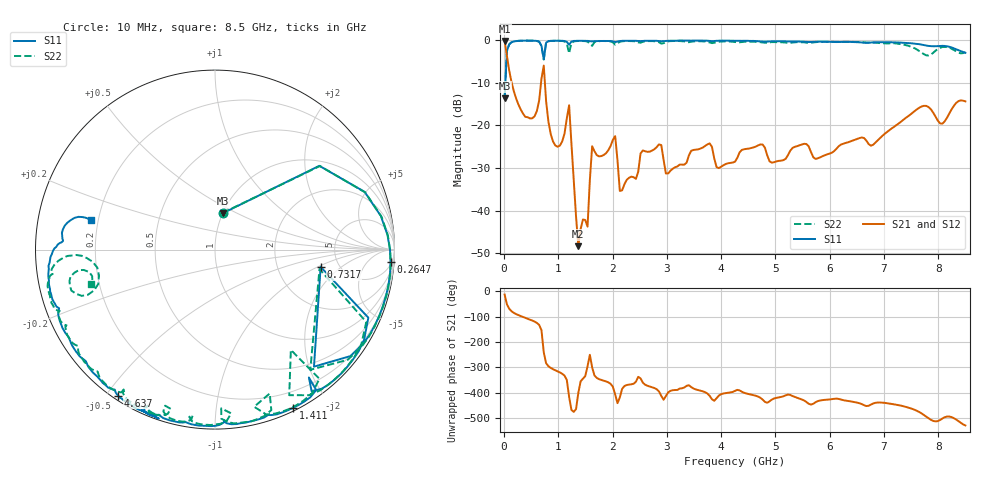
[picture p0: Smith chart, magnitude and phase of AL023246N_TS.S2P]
!AVX CORPORATION
!PN: AL023246N_TS
!DESCRIPTION: AIR CORE INDUCTOR, 246nH, 15 turns
!Agilent Technologies,E5071C,MY46102230,A.09.54
!Date: Mon Sep 03 16:47:05 2012
!Data & Calibration Information:
!Freq	S11:SOLT2(ON)	S21:SOLT2(ON)	S12:SOLT2(ON)	S22:SOLT2(ON)
# Hz S dB R 50
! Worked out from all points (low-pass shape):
!   201 points, 10 MHz to 8.5 GHz, reference 50 ohm
!   highest |S21| = -0.17 dB at 10 MHz (marker M1); lowest = -48.3 dB at 1.368 GHz (marker M2)
!   |S21| within 3 dB of the highest: start of sweep to 47.5 MHz
!   lowest |S11| = -13.7 dB at 10 MHz (marker M3), VSWR 1.52, Z = 50.1 + j21.2 ohm
!   |S11| at or under -10 dB: start of sweep to 23.99 MHz
!   |S22| runs from -13.6 to -0.1 dB; largest |S21 - S12| = 0.0029
!   S11 on the Smith chart (normalised r, x): 10 MHz: 1.00, +0.42; 264.7 MHz: 7, -26; 731.6 MHz: 3.61, -1.08; 1.411 GHz: 0.03, -1.61; 4.637 GHz: 0.02, -0.54; 8.5 GHz: 0.17, +0.12
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1e7  -13.66 77.9  -0.17 -12.6  -0.18 -12.7  -13.62 78.4
9.49e7  -0.98 21.1  -7.12 -68.7  -7.11 -68.7  -0.96 20.9
2.647e8  -0.17 -4.1  -15.11 -93.9  -15.09 -94.0  -0.15 -4.7
5.6185e8  -0.14 -28.3  -17.86 -119.2  -17.85 -119.3  -0.13 -29.6
6.892e8  -1.37 -49.8  -9.04 -153.1  -9.03 -153.2  -1.37 -51.6
7.3165e8  -4.49 -9.3  -5.97 119.2  -5.96 119.2  -4.55 -10.6
9.439e8  -0.13 -41.9  -24.70 48.7  -24.70 48.5  -0.13 -44.2
1.1986e9  -1.07 -53.7  -15.28 -56.4  -15.29 -56.5  -3.09 -52.9
1.3684e9  -0.15 -61.7  -48.34 -40.3  -48.23 -39.4  -0.19 -62.3
1.41085e9  -0.15 -63.7  -44.30 5.1  -44.20 2.8  -0.18 -64.7
1.4533e9  -0.15 -65.7  -42.08 15.2  -42.10 16.2  -0.20 -67.2
1.5382e9  -0.17 -69.4  -43.75 64.5  -43.96 64.9  -0.33 -72.7
1.6231e9  -0.29 -72.2  -24.89 59.7  -24.90 59.5  -1.33 -69.2
2.0476e9  -0.44 -87.0  -22.51 -47.1  -22.51 -47.2  -1.06 -87.8
2.1325e9  -0.21 -88.4  -35.37 -58.5  -35.41 -58.5  -0.36 -86.2
2.85415e9  -0.20 -107.9  -24.46 -34.9  -24.46 -35.1  -0.48 -107.7
2.9815e9  -0.17 -109.8  -31.28 -53.4  -31.32 -53.6  -0.42 -106.1
4.255e9  -0.14 -118.3  -28.52 -32.9  -28.54 -32.9  -0.43 -133.1
4.63705e9  -0.21 -123.5  -24.97 -51.9  -24.98 -52.0  -0.40 -141.5
5.6983e9  -0.41 -140.2  -27.48 -83.2  -27.53 -83.0  -0.54 -158.8
7.09915e9  -0.49 -167.7  -21.12 -82.6  -21.14 -82.6  -0.74 -171.7
8.5e9  -2.95 166.4  -14.37 -169.0  -14.37 -169.1  -2.87 -164.6
